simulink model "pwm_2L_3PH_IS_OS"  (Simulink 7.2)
settings: Solver=ode3  SolverMode=SingleTasking  StartTime=0.0  StopTime=0.1  FixedStep=1e-6  MaxStep=1e-4  RelTol=1e-3
PreLoadFcn:
  | INIT_PWM_2L

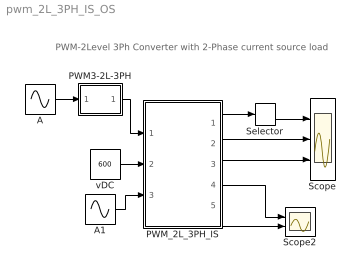
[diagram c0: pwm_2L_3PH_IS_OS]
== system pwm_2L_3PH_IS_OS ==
  note: PWM-2Level 3Ph Converter with 2-Phase current source load
  A : Sin  Amplitude=.9  Frequency=2*pi*50  Phase="[0  -2*pi/3  -4*pi/3]"  SampleTime=0
  A1 : Sin  Amplitude=400  Frequency=2*pi*50  Phase="[0  -2*pi/3 ]"  SampleTime=0
  PWM3-2L-3PH : Subsystem  mask(PWM3-2L-3PH){FT=900, PHT=0, DT=1e-6}
      mask prompts: FT "Triangular Frequency"; PHT "Trian. Phase Angle (Degree)"; DT "Dead Time"
      mask help: Pulse Width Modulation for 3 Phase Converter
  PWM_2L_3PH_IS : Subsystem
  Scope : Scope  NumInputPorts=3
  Scope2 : Scope  NumInputPorts=2
  Selector : Selector  InputPortWidth=3  IndexOptions=Index vector (dialog)  Indices=[1 ]  OutputSizes=1
  vDC : Constant  Value=600  OutDataType=sfix(16)  OutScaling=2^0
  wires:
  A/1 -> PWM3-2L-3PH/1(In4)
  PWM_2L_3PH_IS/1(vABC) -> Selector/1
  PWM_2L_3PH_IS/2(iABC) -> Scope/2
  PWM_2L_3PH_IS/3(vAB) -> Scope/3
  PWM_2L_3PH_IS/4(iT1,iD1,vT1) -> Scope2/1
  PWM_2L_3PH_IS/5(iDC) -> Scope2/2
  vDC/1 -> PWM_2L_3PH_IS/2(vDC)
  A1/1 -> PWM_2L_3PH_IS/3(I_AB)
  PWM3-2L-3PH/1(Out1) -> PWM_2L_3PH_IS/1(Sw)
  Selector/1 -> Scope/1

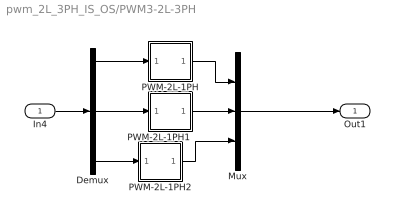
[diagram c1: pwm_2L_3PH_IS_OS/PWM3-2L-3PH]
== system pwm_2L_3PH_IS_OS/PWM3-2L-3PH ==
  In4 : Inport
  Demux : Demux  Outputs=3
  Mux : Mux  Inputs=3
  PWM-2L-1PH : Subsystem  mask(PWM-2L-1PH){FT=FT, PHT=PHT, DT=DT}
      mask prompts: FT "Triangular Frequency"; PHT "Trian. Phase Angle (Degree)"; DT "Dead Time"
      mask help: Pulse Width Modulation for 1 Phase Converter
  PWM-2L-1PH1 : Subsystem  mask(PWM-2L-1PH){FT=FT, PHT=PHT, DT=DT}
      mask prompts: FT "Triangular Frequency"; PHT "Trian. Phase Angle (Degree)"; DT "Dead Time"
      mask help: Pulse Width Modulation for 1 Phase Converter
  PWM-2L-1PH2 : Subsystem  mask(PWM-2L-1PH){FT=FT, PHT=PHT, DT=DT}
      mask prompts: FT "Triangular Frequency"; PHT "Trian. Phase Angle (Degree)"; DT "Dead Time"
      mask help: Pulse Width Modulation for 1 Phase Converter
  Out1 : Outport
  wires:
  In4/1 -> Demux/1
  Demux/3 -> PWM-2L-1PH2/1(In1)
  Demux/2 -> PWM-2L-1PH1/1(In1)
  Demux/1 -> PWM-2L-1PH/1(In1)
  PWM-2L-1PH1/1(Out1) -> Mux/2
  PWM-2L-1PH/1(Out1) -> Mux/1
  PWM-2L-1PH2/1(Out1) -> Mux/3
  Mux/1 -> Out1/1

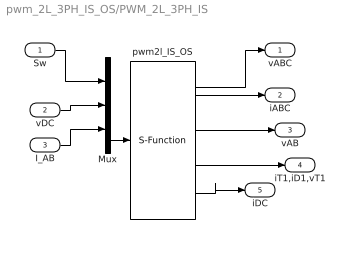
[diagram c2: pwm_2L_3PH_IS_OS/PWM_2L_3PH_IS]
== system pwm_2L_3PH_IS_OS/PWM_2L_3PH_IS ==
  Sw : Inport  OutDataType=sfix(16)  OutScaling=2^0
  vDC : Inport  Port=2  OutDataType=sfix(16)  OutScaling=2^0
  I_AB : Inport  Port=3  OutDataType=sfix(16)  OutScaling=2^0
  Mux : Mux  Inputs="[6  1  2]"
  pwm2l_IS_OS : S-Function  FunctionName=s_pwm_2L_3PH_IS_OS  Parameters=0  EnableBusSupport=off
  vABC : Outport  OutDataType=sfix(16)  OutScaling=2^0
  iABC : Outport  Port=2  OutDataType=sfix(16)  OutScaling=2^0
  vAB : Outport  Port=3  OutDataType=sfix(16)  OutScaling=2^0
  iT1,iD1,vT1 : Outport  Port=4  OutDataType=sfix(16)  OutScaling=2^0
  iDC : Outport  Port=5  OutDataType=sfix(16)  OutScaling=2^0
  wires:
  Sw/1 -> Mux/1
  vDC/1 -> Mux/2
  Mux/1 -> pwm2l_IS_OS/1
  I_AB/1 -> Mux/3
  pwm2l_IS_OS/4 -> iT1,iD1,vT1/1
  pwm2l_IS_OS/1 -> vABC/1
  pwm2l_IS_OS/2 -> iABC/1
  pwm2l_IS_OS/3 -> vAB/1
  pwm2l_IS_OS/5 -> iDC/1

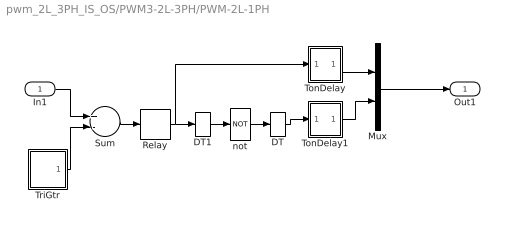
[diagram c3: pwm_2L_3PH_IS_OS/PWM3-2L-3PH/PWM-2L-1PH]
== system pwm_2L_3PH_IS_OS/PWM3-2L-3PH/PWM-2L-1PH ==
  In1 : Inport
  DT : DataTypeConversion
  DT1 : DataTypeConversion
  Mux : Mux  Inputs=2
  Relay : Relay
  Sum : Sum  Inputs=+-
  TonDelay : Subsystem  mask(TonDelay){DT=DT}
      mask prompts: DT "Dead Time"
      mask help: Turn on dead time to protect against short circuit of the converter leg
  TonDelay1 : Subsystem  mask(TonDelay){DT=DT}
      mask prompts: DT "Dead Time"
      mask help: Turn on dead time to protect against short circuit of the converter leg
  TriGtr : Subsystem  mask(TriGtr){T=1/FT, Td=PHT/FT/360}
      mask prompts: T "Period Time"; Td "Time Delay"
      mask help: Triangular Wave Generator with variable time delay
  not : Logic  Operator=NOT  Inputs=1
  Out1 : Outport  InitialOutput=0
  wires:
  Mux/1 -> Out1/1
  TonDelay/1(s1d) -> Mux/1
  Relay/1 -> TonDelay/1(s1), DT1/1
  TonDelay1/1(s1d) -> Mux/2
  not/1 -> DT/1
  Sum/1 -> Relay/1
  TriGtr/1(O) -> Sum/2
  In1/1 -> Sum/1
  DT/1 -> TonDelay1/1(s1)
  DT1/1 -> not/1

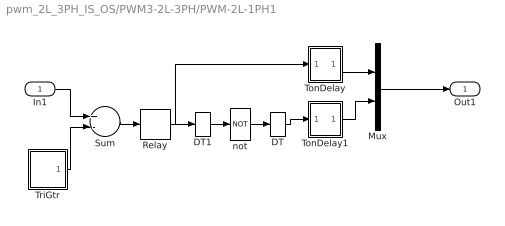
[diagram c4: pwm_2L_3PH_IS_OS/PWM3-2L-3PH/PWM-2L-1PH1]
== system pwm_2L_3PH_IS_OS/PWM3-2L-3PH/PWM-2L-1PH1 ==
  In1 : Inport
  DT : DataTypeConversion
  DT1 : DataTypeConversion
  Mux : Mux  Inputs=2
  Relay : Relay
  Sum : Sum  Inputs=+-
  TonDelay : Subsystem  mask(TonDelay){DT=DT}
      mask prompts: DT "Dead Time"
      mask help: Turn on dead time to protect against short circuit of the converter leg
  TonDelay1 : Subsystem  mask(TonDelay){DT=DT}
      mask prompts: DT "Dead Time"
      mask help: Turn on dead time to protect against short circuit of the converter leg
  TriGtr : Subsystem  mask(TriGtr){T=1/FT, Td=PHT/FT/360}
      mask prompts: T "Period Time"; Td "Time Delay"
      mask help: Triangular Wave Generator with variable time delay
  not : Logic  Operator=NOT  Inputs=1
  Out1 : Outport  InitialOutput=0
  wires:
  DT1/1 -> not/1
  DT/1 -> TonDelay1/1(s1)
  In1/1 -> Sum/1
  TriGtr/1(O) -> Sum/2
  Sum/1 -> Relay/1
  not/1 -> DT/1
  TonDelay1/1(s1d) -> Mux/2
  Relay/1 -> DT1/1, TonDelay/1(s1)
  TonDelay/1(s1d) -> Mux/1
  Mux/1 -> Out1/1

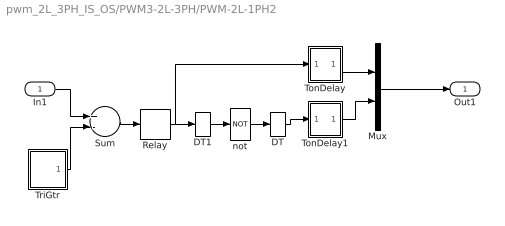
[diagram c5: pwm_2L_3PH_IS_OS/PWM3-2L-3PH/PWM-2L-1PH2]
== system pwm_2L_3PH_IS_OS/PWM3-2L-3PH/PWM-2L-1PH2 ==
  In1 : Inport
  DT : DataTypeConversion
  DT1 : DataTypeConversion
  Mux : Mux  Inputs=2
  Relay : Relay
  Sum : Sum  Inputs=+-
  TonDelay : Subsystem  mask(TonDelay){DT=DT}
      mask prompts: DT "Dead Time"
      mask help: Turn on dead time to protect against short circuit of the converter leg
  TonDelay1 : Subsystem  mask(TonDelay){DT=DT}
      mask prompts: DT "Dead Time"
      mask help: Turn on dead time to protect against short circuit of the converter leg
  TriGtr : Subsystem  mask(TriGtr){T=1/FT, Td=PHT/FT/360}
      mask prompts: T "Period Time"; Td "Time Delay"
      mask help: Triangular Wave Generator with variable time delay
  not : Logic  Operator=NOT  Inputs=1
  Out1 : Outport  InitialOutput=0
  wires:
  Mux/1 -> Out1/1
  TonDelay/1(s1d) -> Mux/1
  Relay/1 -> TonDelay/1(s1), DT1/1
  TonDelay1/1(s1d) -> Mux/2
  not/1 -> DT/1
  Sum/1 -> Relay/1
  TriGtr/1(O) -> Sum/2
  In1/1 -> Sum/1
  DT/1 -> TonDelay1/1(s1)
  DT1/1 -> not/1

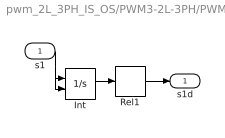
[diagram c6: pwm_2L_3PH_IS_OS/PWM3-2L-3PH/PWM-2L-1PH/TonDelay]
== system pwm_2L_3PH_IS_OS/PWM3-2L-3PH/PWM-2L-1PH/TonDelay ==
  s1 : Inport
  Int : Integrator  ExternalReset=falling
  Rel1 : Relay  OnSwitchValue=DT
  s1d : Outport  InitialOutput=0
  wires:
  Rel1/1 -> s1d/1
  s1/1 -> Int/1, Int/2
  Int/1 -> Rel1/1

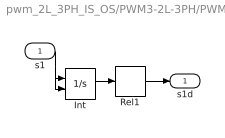
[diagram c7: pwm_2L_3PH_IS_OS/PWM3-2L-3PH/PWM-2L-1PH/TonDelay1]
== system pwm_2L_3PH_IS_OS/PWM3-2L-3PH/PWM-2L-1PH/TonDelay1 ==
  s1 : Inport
  Int : Integrator  ExternalReset=falling
  Rel1 : Relay  OnSwitchValue=DT
  s1d : Outport  InitialOutput=0
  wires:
  Rel1/1 -> s1d/1
  s1/1 -> Int/1, Int/2
  Int/1 -> Rel1/1

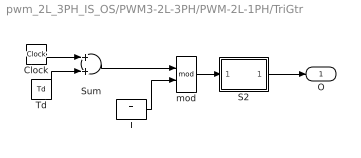
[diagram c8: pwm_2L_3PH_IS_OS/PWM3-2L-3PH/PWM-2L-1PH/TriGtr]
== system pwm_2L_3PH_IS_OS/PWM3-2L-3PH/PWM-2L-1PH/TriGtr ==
  Clock : Clock
  S2 : Subsystem
  Sum : Sum
  T : Constant  Value=T
  Td : Constant  Value=Td
  mod : Math  Operator=mod
  O : Outport  InitialOutput=0
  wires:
  Td/1 -> Sum/2
  Sum/1 -> mod/1
  T/1 -> mod/2
  Clock/1 -> Sum/1
  S2/1(O1) -> O/1
  mod/1 -> S2/1(I1)

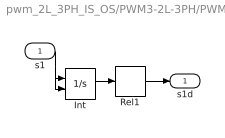
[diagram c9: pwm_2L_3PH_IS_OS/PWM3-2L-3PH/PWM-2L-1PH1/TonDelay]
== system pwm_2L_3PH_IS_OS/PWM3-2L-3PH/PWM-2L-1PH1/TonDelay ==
  s1 : Inport
  Int : Integrator  ExternalReset=falling
  Rel1 : Relay  OnSwitchValue=DT
  s1d : Outport  InitialOutput=0
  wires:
  Int/1 -> Rel1/1
  s1/1 -> Int/2, Int/1
  Rel1/1 -> s1d/1

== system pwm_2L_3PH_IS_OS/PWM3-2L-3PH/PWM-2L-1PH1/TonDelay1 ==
  s1 : Inport
  Int : Integrator  ExternalReset=falling
  Rel1 : Relay  OnSwitchValue=DT
  s1d : Outport  InitialOutput=0
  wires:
  Int/1 -> Rel1/1
  s1/1 -> Int/2, Int/1
  Rel1/1 -> s1d/1

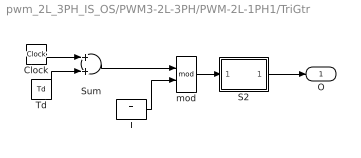
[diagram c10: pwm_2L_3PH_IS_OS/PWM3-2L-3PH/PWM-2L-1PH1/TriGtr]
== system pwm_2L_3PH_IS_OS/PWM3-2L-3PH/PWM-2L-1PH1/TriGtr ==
  Clock : Clock
  S2 : Subsystem
  Sum : Sum
  T : Constant  Value=T
  Td : Constant  Value=Td
  mod : Math  Operator=mod
  O : Outport  InitialOutput=0
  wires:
  mod/1 -> S2/1(I1)
  S2/1(O1) -> O/1
  Clock/1 -> Sum/1
  T/1 -> mod/2
  Sum/1 -> mod/1
  Td/1 -> Sum/2

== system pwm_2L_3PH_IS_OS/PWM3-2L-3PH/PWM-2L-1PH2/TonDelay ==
  s1 : Inport
  Int : Integrator  ExternalReset=falling
  Rel1 : Relay  OnSwitchValue=DT
  s1d : Outport  InitialOutput=0
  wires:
  Rel1/1 -> s1d/1
  s1/1 -> Int/1, Int/2
  Int/1 -> Rel1/1

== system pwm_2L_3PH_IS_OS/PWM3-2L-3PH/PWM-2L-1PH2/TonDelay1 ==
  s1 : Inport
  Int : Integrator  ExternalReset=falling
  Rel1 : Relay  OnSwitchValue=DT
  s1d : Outport  InitialOutput=0
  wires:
  Rel1/1 -> s1d/1
  s1/1 -> Int/1, Int/2
  Int/1 -> Rel1/1

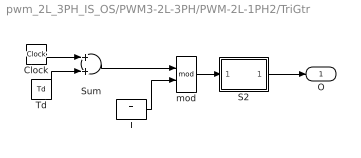
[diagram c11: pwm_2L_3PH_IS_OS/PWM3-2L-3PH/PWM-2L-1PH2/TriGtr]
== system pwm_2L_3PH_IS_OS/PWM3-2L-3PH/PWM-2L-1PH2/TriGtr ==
  Clock : Clock
  S2 : Subsystem
  Sum : Sum
  T : Constant  Value=T
  Td : Constant  Value=Td
  mod : Math  Operator=mod
  O : Outport  InitialOutput=0
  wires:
  Td/1 -> Sum/2
  Sum/1 -> mod/1
  T/1 -> mod/2
  Clock/1 -> Sum/1
  S2/1(O1) -> O/1
  mod/1 -> S2/1(I1)

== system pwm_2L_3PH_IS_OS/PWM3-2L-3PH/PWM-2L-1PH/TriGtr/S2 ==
  I1 : Inport
  Fcn : Fcn  Expr="(u* (u <=T/4) * 4/T)   +  (  (u > T/4) && ( u <=3*T/4) )* ( 1 - (u-T/4) *4/T )   +  ( (u > 3*T/4)&& (u<=T)) * ( ((u -3*T/4)* 4/T )-1 )"
  O1 : Outport
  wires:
  I1/1 -> Fcn/1
  Fcn/1 -> O1/1

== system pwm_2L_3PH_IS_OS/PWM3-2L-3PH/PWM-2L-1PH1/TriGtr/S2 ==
  I1 : Inport
  Fcn : Fcn  Expr="(u* (u <=T/4) * 4/T)   +  (  (u > T/4) && ( u <=3*T/4) )* ( 1 - (u-T/4) *4/T )   +  ( (u > 3*T/4)&& (u<=T)) * ( ((u -3*T/4)* 4/T )-1 )"
  O1 : Outport
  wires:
  Fcn/1 -> O1/1
  I1/1 -> Fcn/1

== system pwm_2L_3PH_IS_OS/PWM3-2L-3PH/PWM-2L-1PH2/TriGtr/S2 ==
  I1 : Inport
  Fcn : Fcn  Expr="(u* (u <=T/4) * 4/T)   +  (  (u > T/4) && ( u <=3*T/4) )* ( 1 - (u-T/4) *4/T )   +  ( (u > 3*T/4)&& (u<=T)) * ( ((u -3*T/4)* 4/T )-1 )"
  O1 : Outport
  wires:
  I1/1 -> Fcn/1
  Fcn/1 -> O1/1
